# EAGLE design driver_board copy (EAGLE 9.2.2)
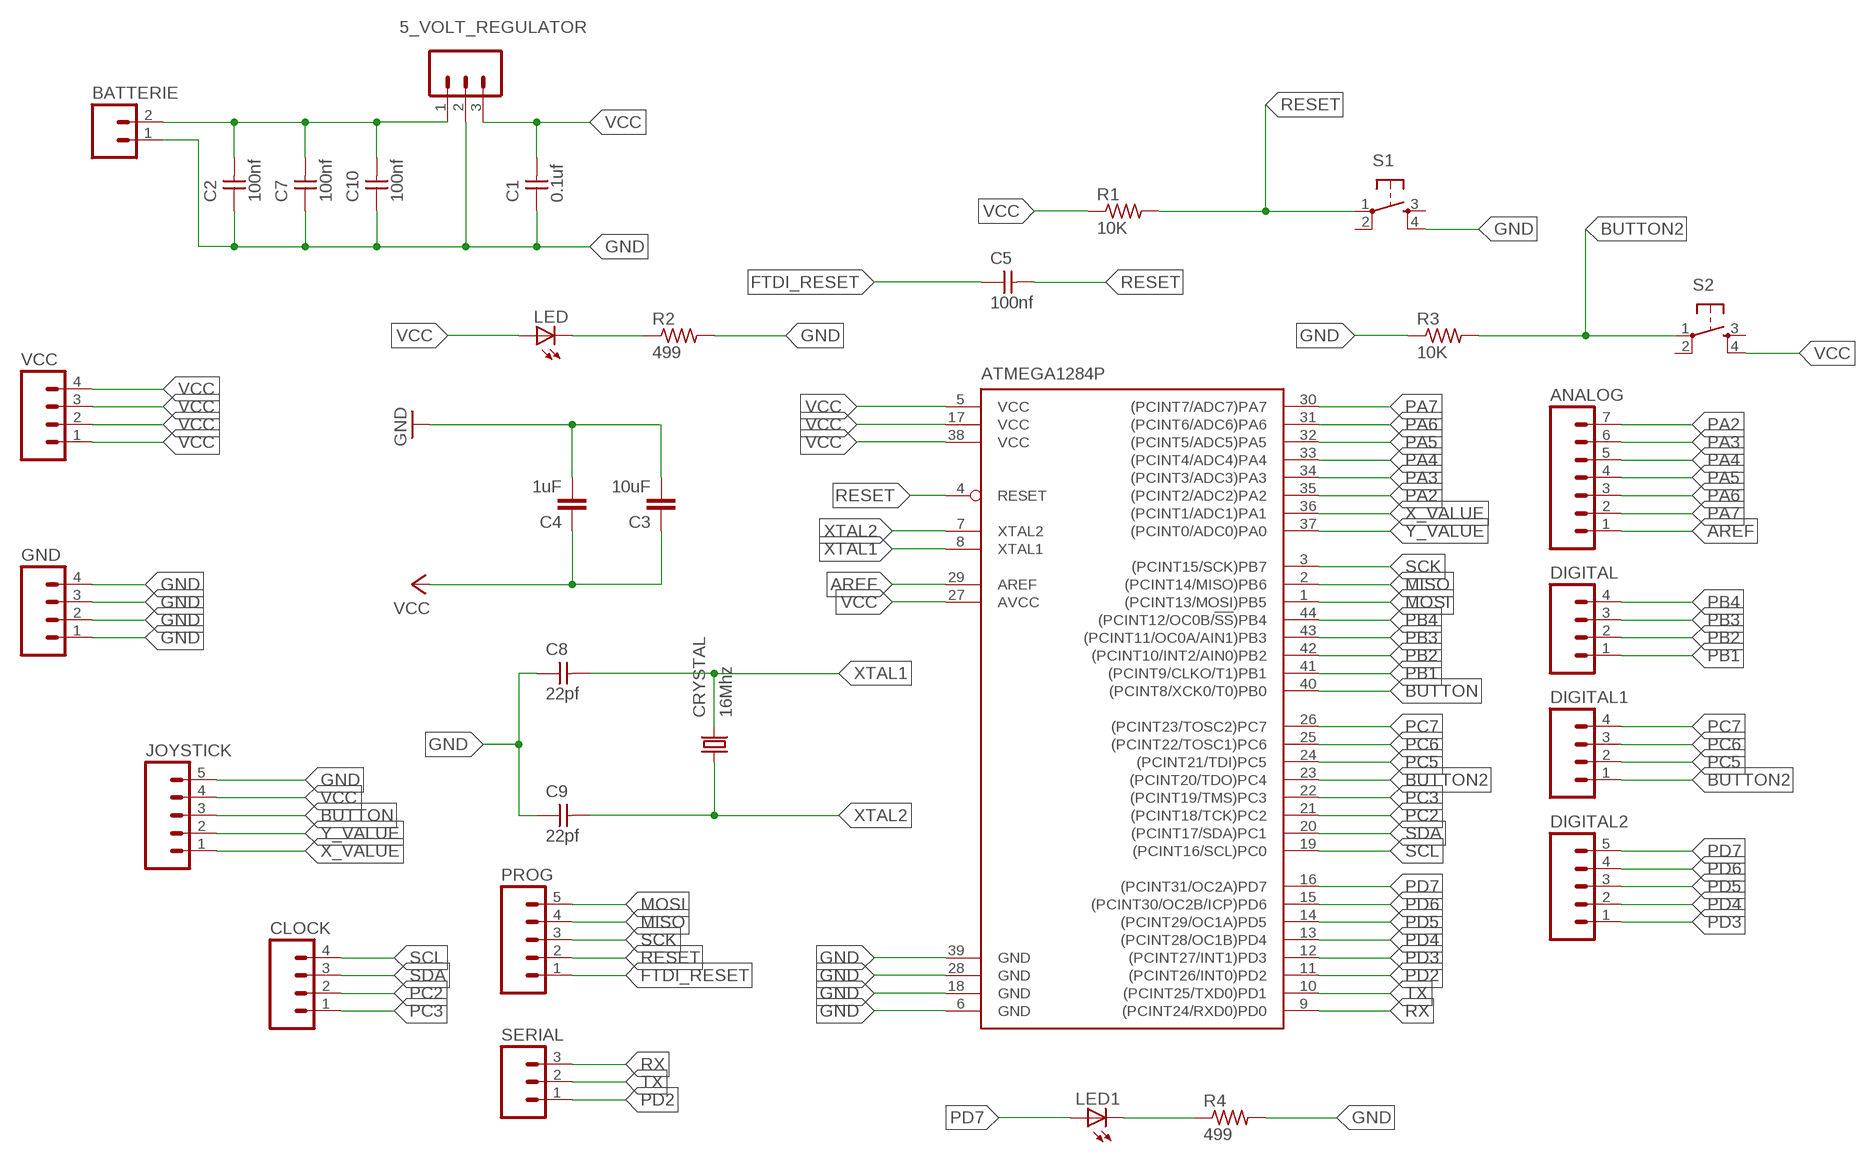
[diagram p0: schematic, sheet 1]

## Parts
5_VOLT_REGULATOR  M03  [03P]
ANALOG  M07  [07P]
ATMEGA1284P  ATMEGA644A  [TQFP44]
BATTERIE  M02  [02P]
C1  0.1uf  UNPOLARIZED_CAPACITOR1206  [1206]
C2  100nf  UNPOLARIZED_CAPACITOR1206  [1206]
C3  10uF  CAP1206  [1206]
C4  1uF  CAP1206  [1206]
C5  100nf  UNPOLARIZED_CAPACITOR1206  [1206]
C7  100nf  UNPOLARIZED_CAPACITOR1206  [1206]
C8  22pf  UNPOLARIZED_CAPACITOR1206  [1206]
C9  22pf  UNPOLARIZED_CAPACITOR1206  [1206]
C10  100nf  UNPOLARIZED_CAPACITOR1206  [1206]
CLOCK  M04  [04P]
CRYSTAL  16Mhz  KX-12B  [6.0X3.5_2]
DIGITAL  M04  [04P]
DIGITAL1  M04  [04P]
DIGITAL2  M05  [05P]
GND  M04  [04P]
JOYSTICK  M05  [05P]
LED  LED1206  [1206]
LED1  LED1206  [1206]
PROG  M05  [05P]
R1  10K  RESISTOR1206  [1206]
R2  499  RESISTOR1206  [1206]
R3  10K  RESISTOR1206  [1206]
R4  499  RESISTOR1206  [1206]
S1  6MM_SWITCH6MM_SWITCH  [6MM_SWITCH]
S2  6MM_SWITCH6MM_SWITCH  [6MM_SWITCH]
SERIAL  M03  [03P]
VCC  M04  [04P]

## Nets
AREF: ANALOG.1 ATMEGA1284P.29(AREF)
BUTTON: ATMEGA1284P.40((PCINT8/XCK0/T0)PB0) JOYSTICK.3
BUTTON2: ATMEGA1284P.23((PCINT20/TDO)PC4) DIGITAL1.1 R3.2 S2.1(P)
FTDI_RESET: C5.1 PROG.1
GND: 5_VOLT_REGULATOR.2 ATMEGA1284P.6(GND) ATMEGA1284P.18(GND) ATMEGA1284P.28(GND) ATMEGA1284P.39(GND) BATTERIE.1 C1.1 C2.1 C3.2 C4.2 C7.1 C8.1 C9.1 C10.1 GND.1 GND.2 GND.3 GND.4 JOYSTICK.5 R2.2 R3.1 R4.2 S1.4(S1)
MISO: ATMEGA1284P.2((PCINT14/MISO)PB6) PROG.4
MOSI: ATMEGA1284P.1((PCINT13/MOSI)PB5) PROG.5
MOTOR_VCC: 5_VOLT_REGULATOR.1 BATTERIE.2 C2.2 C7.2 C10.2
N$1: LED.2(C) R2.1
N$2: LED1.2(C) R4.1
PA2: ANALOG.7 ATMEGA1284P.35((PCINT2/ADC2)PA2)
PA3: ANALOG.6 ATMEGA1284P.34((PCINT3/ADC3)PA3)
PA4: ANALOG.5 ATMEGA1284P.33((PCINT4/ADC4)PA4)
PA5: ANALOG.4 ATMEGA1284P.32((PCINT5/ADC5)PA5)
PA6: ANALOG.3 ATMEGA1284P.31((PCINT6/ADC6)PA6)
PA7: ANALOG.2 ATMEGA1284P.30((PCINT7/ADC7)PA7)
PB1: ATMEGA1284P.41((PCINT9/CLKO/T1)PB1) DIGITAL.1
PB2: ATMEGA1284P.42((PCINT10/INT2/AIN0)PB2) DIGITAL.2
PB3: ATMEGA1284P.43((PCINT11/OC0A/AIN1)PB3) DIGITAL.3
PB4: ATMEGA1284P.44((PCINT12/OC0B/!SS!)PB4) DIGITAL.4
PC2: ATMEGA1284P.21((PCINT18/TCK)PC2) CLOCK.2
PC3: ATMEGA1284P.22((PCINT19/TMS)PC3) CLOCK.1
PC5: ATMEGA1284P.24((PCINT21/TDI)PC5) DIGITAL1.2
PC6: ATMEGA1284P.25((PCINT22/TOSC1)PC6) DIGITAL1.3
PC7: ATMEGA1284P.26((PCINT23/TOSC2)PC7) DIGITAL1.4
PD2: ATMEGA1284P.11((PCINT26/INT0)PD2) SERIAL.1
PD3: ATMEGA1284P.12((PCINT27/INT1)PD3) DIGITAL2.1
PD4: ATMEGA1284P.13((PCINT28/OC1B)PD4) DIGITAL2.2
PD5: ATMEGA1284P.14((PCINT29/OC1A)PD5) DIGITAL2.3
PD6: ATMEGA1284P.15((PCINT30/OC2B/ICP)PD6) DIGITAL2.4
PD7: ATMEGA1284P.16((PCINT31/OC2A)PD7) DIGITAL2.5 LED1.1(A)
RESET: ATMEGA1284P.4(RESET) C5.2 PROG.2 R1.2 S1.1(P)
RX: ATMEGA1284P.9((PCINT24/RXD0)PD0) SERIAL.3
SCK: ATMEGA1284P.3((PCINT15/SCK)PB7) PROG.3
SCL: ATMEGA1284P.19((PCINT16/SCL)PC0) CLOCK.4
SDA: ATMEGA1284P.20((PCINT17/SDA)PC1) CLOCK.3
TX: ATMEGA1284P.10((PCINT25/TXD0)PD1) SERIAL.2
VCC: 5_VOLT_REGULATOR.3 ATMEGA1284P.5(VCC) ATMEGA1284P.17(VCC) ATMEGA1284P.27(AVCC) ATMEGA1284P.38(VCC) C1.2 C3.1 C4.1 JOYSTICK.4 LED.1(A) R1.1 S2.4(S1) VCC.1 VCC.2 VCC.3 VCC.4
X_VALUE: ATMEGA1284P.36((PCINT1/ADC1)PA1) JOYSTICK.1
XTAL1: ATMEGA1284P.8(XTAL1) C8.2 CRYSTAL.2
XTAL2: ATMEGA1284P.7(XTAL2) C9.2 CRYSTAL.1
Y_VALUE: ATMEGA1284P.37((PCINT0/ADC0)PA0) JOYSTICK.2
Unconnected: S1.2(P1) S1.3(S) S2.2(P1) S2.3(S)

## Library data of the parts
5_VOLT_REGULATOR SERIAL = con-amp-quick:M03: AMP QUICK CONNECTOR; OC_FARNELL: unknown; OC_NEWARK: unknown
ANALOG = con-amp-quick:M07: AMP QUICK CONNECTOR; OC_FARNELL: unknown; OC_NEWARK: unknown
ATMEGA1284P = atmel:ATMEGA644: 8-bit Microcontroller with 64K Bytes In-System Programmable Flash Source: http://www.atmel.com/dyn/resources/prod_documents/doc2593.pdf; MPN: ATMEGA644PV-10AU; OC_FARNELL: 1455123; OC_NEWARK: 58M3748
BATTERIE = con-amp-quick:M02: AMP QUICK CONNECTOR; OC_FARNELL: unknown; OC_NEWARK: unknown
C1 C2 C5 C7-C10 = FAB_Hello:UNPOLARIZED_CAPACITOR: unpolarized_capacitor
C3 C4 = 01_SparkFun:CAP: Capacitor
CLOCK DIGITAL DIGITAL1 GND VCC = con-amp-quick:M04: AMP QUICK CONNECTOR; OC_FARNELL: unknown; OC_NEWARK: unknown
CRYSTAL = crystal-geyer_V1_0:KX
DIGITAL2 JOYSTICK PROG = con-amp-quick:M05: AMP QUICK CONNECTOR; OC_FARNELL: unknown; OC_NEWARK: unknown
LED LED1 = FAB_Hello:LED
R1-R4 = FAB_Hello:RESISTOR
S1 S2 = FAB_Hello:6MM_SWITCH: OMRON SWITCH

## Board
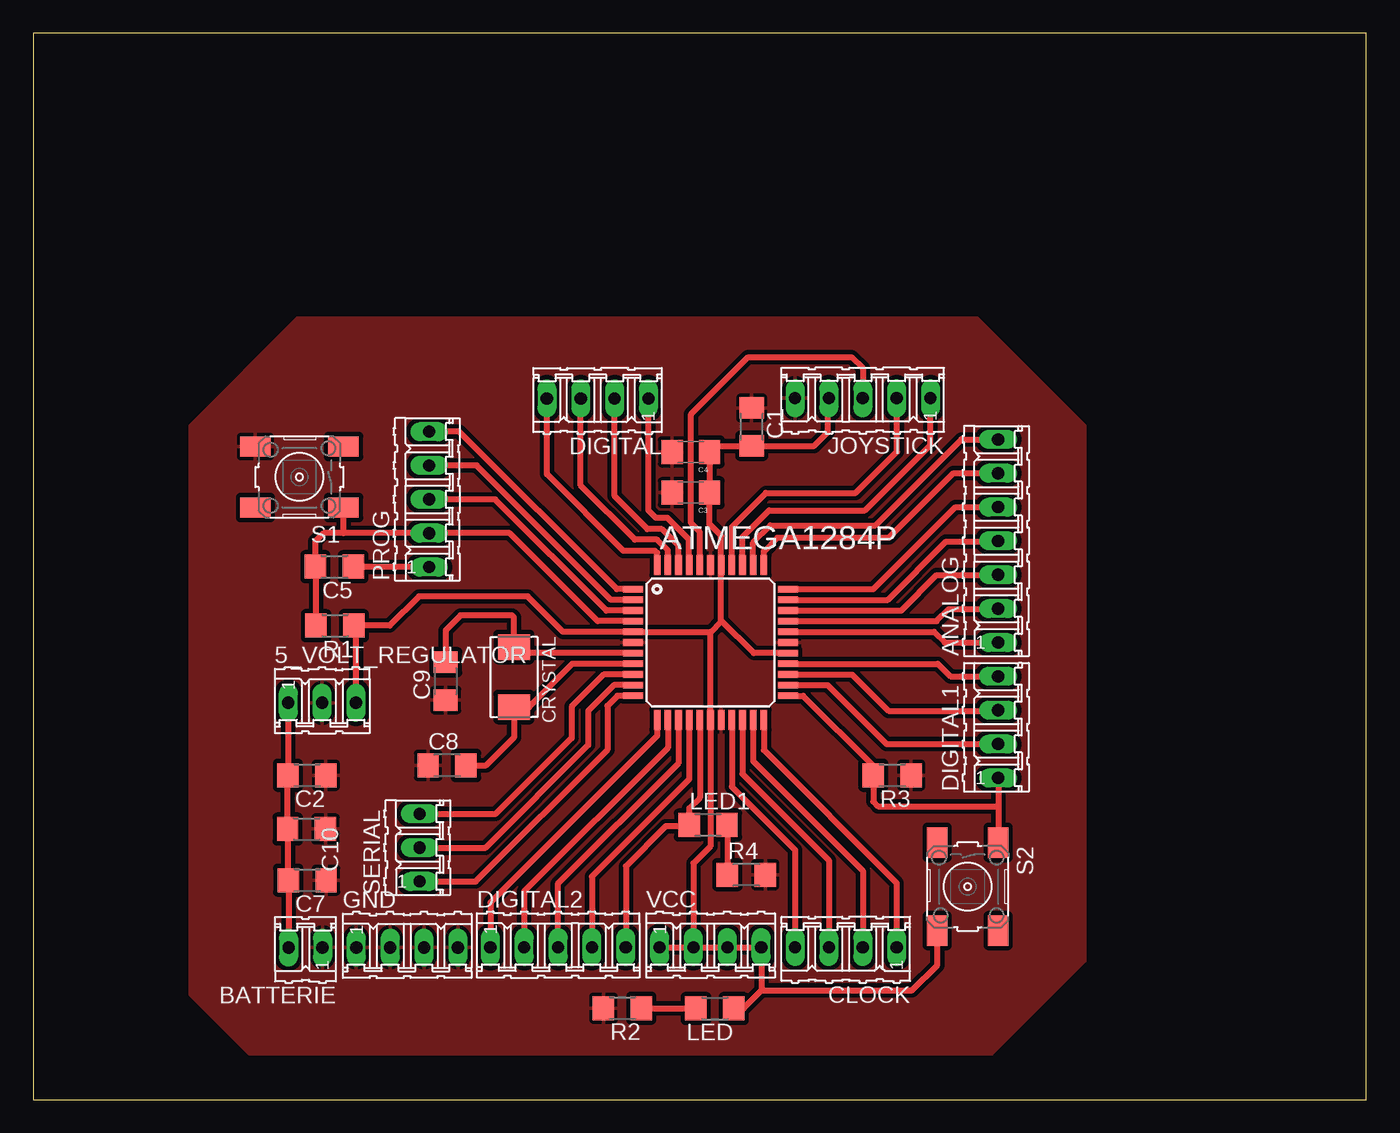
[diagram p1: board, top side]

Size 100 x 80 mm. Coordinates in mm from the lower left corner, seen from the top.
Outline: 0,0 100,0 100,80 0,80 0,0
Copper layers (1*16): Top 0.035mm / dielectric 1.5mm / Bottom 0.035mm
Design rules "default": minimum track width 6mil, minimum drill 0.35mm, track to track 6mil, track to pad 6mil, pad to pad 6mil, via to via 6mil, smd to smd 6mil, copper to edge 40mil, drill to drill 6mil, minimum pad ring 10mil, minimum via ring 8mil, stop-mask expansion 4mil, vias tented up to drill 0mil, thermal gap 10mil

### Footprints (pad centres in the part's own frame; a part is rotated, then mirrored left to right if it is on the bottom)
03P = drill 0.914 long: 1 -2.54,0; 2 0,0; 3 2.54,0
07P = drill 0.914 long: 1 -7.62,0; 2 -5.08,0; 3 -2.54,0; 4 0,0; 5 2.54,0; 6 5.08,0; 7 7.62,0
TQFP44 = smd 1.5 x 0.5: 1 -5.8,4; 2 -5.8,3.2; 3 -5.8,2.4; 4 -5.8,1.6; 5 -5.8,0.8; 6 -5.8,0; 7 -5.8,-0.8; 8 -5.8,-1.6; 9 -5.8,-2.4; 10 -5.8,-3.2; 11 -5.8,-4; 23 5.8,-4; 24 5.8,-3.2; 25 5.8,-2.4; 26 5.8,-1.6; 27 5.8,-0.8; 28 5.8,0; 29 5.8,0.8; 30 5.8,1.6; 31 5.8,2.4; 32 5.8,3.2; 33 5.8,4 | smd 0.5 x 1.5: 12 -4,-5.8; 13 -3.2,-5.8; 14 -2.4,-5.8; 15 -1.6,-5.8; 16 -0.8,-5.8; 17 0,-5.8; 18 0.8,-5.8; 19 1.6,-5.8; 20 2.4,-5.8; 21 3.2,-5.8; 22 4,-5.8; 34 4,5.8; 35 3.2,5.8; 36 2.4,5.8; 37 1.6,5.8; 38 0.8,5.8; 39 0,5.8; 40 -0.8,5.8; 41 -1.6,5.8; 42 -2.4,5.8; 43 -3.2,5.8; 44 -4,5.8
02P = drill 0.914 long: 1 -1.27,0; 2 1.27,0
1206 = smd 1.6 x 1.803: 1 -1.422,0; 2 1.422,0
1206' = smd 1.6 x 1.8: 1 -1.4,0; 2 1.4,0
04P = drill 0.914 long: 1 -3.81,0; 2 -1.27,0; 3 1.27,0; 4 3.81,0
6.0X3.5_2 = smd 1.9 x 2.4: 1 -2.25,0; 2 2.25,0
05P = drill 0.914 long: 1 -5.08,0; 2 -2.54,0; 3 0,0; 4 2.54,0; 5 5.08,0
6MM_SWITCH = smd 2.286 x 1.524: 1 -3.302,2.286; 2 3.302,2.286; 3 -3.302,-2.286; 4 3.302,-2.286

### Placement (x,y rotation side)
5_VOLT_REGULATOR  21.67,29.77 0 top
ANALOG  72.39,41.91 90 top
ATMEGA1284P  50.8,34.29 0 top
BATTERIE  20.42,11.4 180 top
C1  53.9,50.47 270 top
C2  20.52,24.33 180 top
C3  10uF  [1206']  49.33,45.54 180 top
C4  1uF  [1206']  49.33,48.59 180 top
C5  22.58,39.98 180 top
C7  20.55,16.46 180 top
C8  31.04,25.07 0 top
C9  30.94,31.39 90 top
C10  20.5,20.29 180 top
CLOCK  60.96,11.43 180 top
CRYSTAL  36.07,31.7 270 top
DIGITAL  42.34,52.6 180 top
DIGITAL1  72.39,27.94 90 top
DIGITAL2  39.37,11.43 0 top
GND  28.04,11.4 0 top
JOYSTICK  62.23,52.63 180 top
LED  51.13,6.83 180 top
LED1  50.62,20.6 0 top
PROG  29.69,45.03 90 top
R1  22.63,35.56 180 top
R2  44.2,6.86 180 top
R3  64.44,24.33 180 top
R4  53.49,16.87 0 top
S1  19.96,46.71 180 top
S2  70.1,15.98 270 top
SERIAL  28.98,18.9 90 top
VCC  50.8,11.43 0 top

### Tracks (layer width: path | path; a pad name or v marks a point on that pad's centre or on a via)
AREF
  Top 0.432: ATMEGA1284P.29 67.58,35.09 68.38,34.29 ANALOG.1
BUTTON
  Top 0.432: ATMEGA1284P.40 49.98,40.12 49.98,42.63 49.35,43.26 49.35,51.44 53.62,55.7 61.39,55.7 62.23,54.86 JOYSTICK.3
BUTTON2
  Top 0.432: ATMEGA1284P.23 57.75,30.29 63.02,25.02 R3.2 63.02,22.35 63.37,22 72.39,22 | DIGITAL1.1 72.39,22 | 72.39,22 S2.1
FTDI_RESET
  Top 0.432: PROG.1 24.03,39.95 C5.1
GND
  pour Top (isolate 0.33): 70.84,58.7 78.94,50.6 78.94,10.36 71.93,3.35 16.21,3.35 11.73,7.82 11.73,50.62 19.81,58.7
MISO
  Top 0.432: ATMEGA1284P.2 43.36,37.49 33.27,47.57 PROG.4
MOSI
  Top 0.432: ATMEGA1284P.1 43.78,38.29 31.95,50.11 PROG.5
MOTOR_VCC
  Top 0.432: BATTERIE.2 19.15,16.43 C7.2 19.13,20.24 C10.2 19.08,24.31 C2.2 19.23,24.46 19.13,24.56 5_VOLT_REGULATOR.1 | BATTERIE.2
N$1
  Top 0.432: R2.1 49.68,6.86 LED.2
N$2
  Top 0.432: LED1.2 52.07,20.57 R4.1
PA2
  Top 0.432: ATMEGA1284P.35 54,41.78 55.3,43.08 63.17,43.08 69.62,49.53 ANALOG.7
PA3
  Top 0.432: ATMEGA1284P.34 54.8,41.13 55.83,42.16 64.21,42.16 69.04,46.99 ANALOG.6
PA4
  Top 0.432: ATMEGA1284P.33 63.03,38.29 69.19,44.45 ANALOG.5
PA5
  Top 0.432: ATMEGA1284P.32 64.11,37.49 68.48,41.86 72.34,41.86 ANALOG.4
PA6
  Top 0.432: ATMEGA1284P.31 65.11,36.69 67.77,39.34 72.36,39.34 ANALOG.3
PA7
  Top 0.432: ATMEGA1284P.30 67.77,35.89 68.68,36.8 72.36,36.8 ANALOG.2
PB1
  Top 0.432: ATMEGA1284P.41 | ATMEGA1284P.41 49.2,42.01 47.57,43.64 46.71,43.64 46.15,44.2 DIGITAL.1
PB2
  Top 0.432: ATMEGA1284P.42 48.4,41.57 47.17,42.8 46.08,42.8 43.61,45.26 DIGITAL.2
PB3
  Top 0.432: ATMEGA1284P.43 47.6,41.22 46.81,42.01 45.14,42.01 41.07,46.08 DIGITAL.3
PB4
  Top 0.432: ATMEGA1284P.44 46.8,41.01 46.63,41.17 44.27,41.17 38.53,46.91 DIGITAL.4
PC2
  Top 0.432: ATMEGA1284P.21 54,25.4 62.23,17.17 CLOCK.2
PC3
  Top 0.432: ATMEGA1284P.22 54.8,26.23 64.77,16.26 CLOCK.1
PC5
  Top 0.432: ATMEGA1284P.24 59.59,31.09 64.01,26.67 DIGITAL1.2
PC6
  Top 0.432: ATMEGA1284P.25 61.43,31.89 64.16,29.16 72.34,29.16 DIGITAL1.3
PC7
  Top 0.432: ATMEGA1284P.26 67.87,32.69 68.81,31.75 DIGITAL1.4
PD2
  Top 0.432: ATMEGA1284P.11 43.83,30.29 43.08,29.54 43.08,26.24 33.2,16.36 SERIAL.1
PD3
  Top 0.432: ATMEGA1284P.12 46.8,27.29 34.29,14.78 DIGITAL2.1
PD4
  Top 0.432: ATMEGA1284P.13 47.6,26.39 36.83,15.62 DIGITAL2.2
PD5
  Top 0.432: ATMEGA1284P.14 48.4,25.23 39.34,16.18 39.34,11.46 DIGITAL2.3
PD6
  Top 0.432: ATMEGA1284P.15 49.2,24.03 41.91,16.74 DIGITAL2.4
PD7
  Top 0.432: ATMEGA1284P.16 50,22.64 49.2,21.84 LED1.1 49.1,20.5 47.45,20.5 44.45,17.5 DIGITAL2.5
RESET
  Top 0.432: R1.2 21.21,39.93 C5.2 21.16,41.86 21.79,42.49 23.27,42.49 | 23.27,42.49 S1.1 | 23.27,42.49 PROG.2 35.74,42.49 42.34,35.89 ATMEGA1284P.4
RX
  Top 0.432: ATMEGA1284P.9 42.79,31.89 40.39,29.49 40.39,27.13 34.7,21.44 SERIAL.3
SCK
  Top 0.432: ATMEGA1284P.3 42.99,36.69 34.65,45.03 PROG.3
SCL
  Top 0.432: ATMEGA1284P.19 52.4,23.47 57.15,18.72 CLOCK.4
SDA
  Top 0.432: ATMEGA1284P.20 53.2,24.45 59.69,17.96 CLOCK.3
TX
  Top 0.432: ATMEGA1284P.10 43.56,31.09 41.63,29.16 41.63,26.59 33.96,18.92 33.93,18.9 SERIAL.2
VCC
  Top 0.432: VCC.2 49.53,17.73 50.8,19 ATMEGA1284P.17 50.8,35.05 50.84,35.09 | VCC.1 VCC.2 | VCC.2 VCC.3 VCC.4 54.63,11.4 54.63,8.18 | 54.63,8.18 | 54.63,8.18 65.91,8.18 67.82,10.08 S2.4 | JOYSTICK.4 59.61,52.55 59.61,50.09 58.57,49.05 C1.2 51.18,49.05 C4.1 C3.1 50.73,43.18 51.6,42.3 ATMEGA1284P.38 51.6,35.95 | ATMEGA1284P.5 45.05,35.14 | 51.6,35.95 51.6,35.85 50.84,35.09 | 51.6,35.95 | ATMEGA1284P.27 54.06,33.49 51.6,35.95 | 54.63,8.18 53.29,6.83 LED.1 | ATMEGA1284P.5 39.74,35.09 37.08,37.74 28.93,37.74 26.75,35.56 R1.1 24.21,35.41 5_VOLT_REGULATOR.3 | ATMEGA1284P.5 50.84,35.09
X_VALUE
  Top 0.432: ATMEGA1284P.36 53.2,42.2 55.19,44.2 62.38,44.2 67.31,49.12 JOYSTICK.1
XTAL1
  Top 0.432: ATMEGA1284P.8 40.44,32.69 37.2,29.45 CRYSTAL.2 36.07,27.15 33.98,25.07 C8.2
XTAL2
  Top 0.432: ATMEGA1284P.7 36.53,33.49 CRYSTAL.1 36.07,36.17 35.92,36.32 32.05,36.32 30.94,35.2 C9.2
Y_VALUE
  Top 0.432: ATMEGA1284P.37 52.4,42.95 54.97,45.52 61.7,45.52 64.8,48.62 64.8,52.6 JOYSTICK.2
